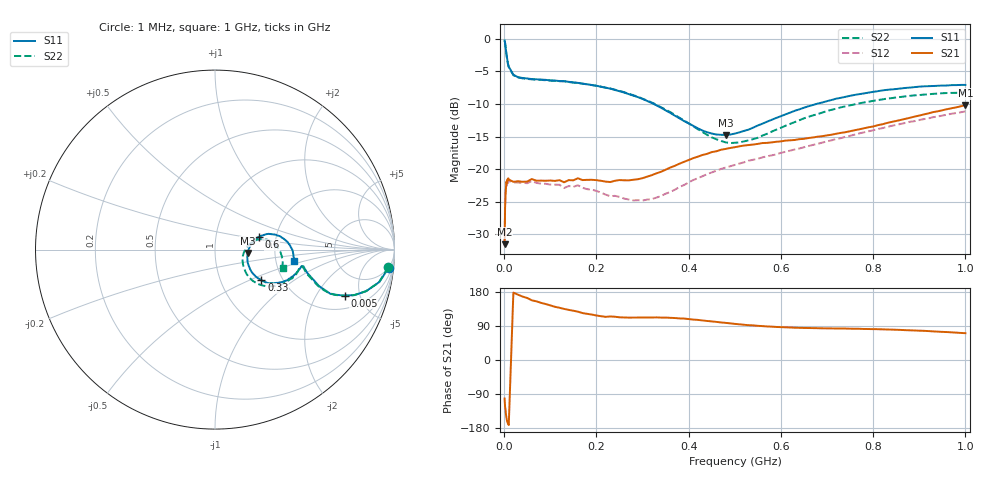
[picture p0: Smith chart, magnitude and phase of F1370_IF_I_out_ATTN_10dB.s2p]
! S-parameters for IF_I+ & IF_I- IDT F1370 DPD Demodulator
! Date Measured:  2015-11-25  RGG
!  Port 1 = Pin 19 = IF_I+
!  Port 2 = Pin 20 = IF_I-
! State: 10 dB attenuation (Gain = Gmax - 10 dB)
! IF Frequency:  1 MHz to 1000 MHz
! RF_INX, RF_INY, IF_Q+, and IF_Q- terminated
! 2300 MHz, 0 dBm signal applied to LO_IN
! Vcc = +5.00 Volts  Icc = approx 275 mA.
! NOTES:  The device was measured on a custom printed circuit evaluation board with individual 50 ohm
!  microstrip lines to the RF and LO pins. The IF outputs are normally connected to balun
!  transformers, which convert the balanced IF output signals to single ended (SE) 50 ohm signals
!  for normal test purposes. For these measurements, to measure the IFI+ and IFI- output SE s-parameters,
!  the chokes associated with the IFI+ and IFI- outputs were removed and a pair of pigtailed
!  50 ohm coaxial lines were soldered to the PCB at these points. 5.00 volt bias was provided
!  to these pins via external bias tees. Data was collected using a calibrated vector
!  network analyzer.  The pigtailed 50 ohm coaxial lines were de-embedded using reference
!  plane extensions. 100 ohm microstrip lines of length 386 mils and 218 mils for the IF_I+ and IF_I-
!  signals, respectively, were de-embedded using Agilent ADS, yielding the reference plane at the IC edge.
!  Only IFI+ and IFI- outputs were measured. IF_Q+ and IF_Q- should be identical.
!  This data is single-ended relative to ports IF_I+ and IF_I- (reference impedance = 50 ohms)
!  Common mode or differential S-parameters may be extracted from this data with a linear simulator.
# mhz S db R 50
! freq  dbS11  angS11  dbS21  angS21  dbS12  angS12  dbS22  angS22
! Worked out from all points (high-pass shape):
!   109 points, 1 MHz to 1 GHz, reference 50 ohm
!   highest |S21| = -10.18 dB at 1 GHz (marker M1); lowest = -31.6 dB at 1 MHz (marker M2)
!   |S21| within 3 dB of the highest: 814.3 MHz to end of sweep
!   lowest |S11| = -14.7 dB at 480 MHz (marker M3), VSWR 1.45, Z = 72.3 - j2.83 ohm
!   |S11| at or under -10 dB: 324.6 MHz to 676.3 MHz (351.8 MHz wide, 70.3 % of centre)
!   |S22| runs from -16.0 to -0.3 dB; largest |S21 - S12| = 0.066
!   S11 on the Smith chart (normalised r, x): 1 MHz: 5, -18; 5 MHz: 2.89, -3.59; 330 MHz: 1.56, -0.59; 600 MHz: 1.63, +0.25; 1 GHz: 2.52, -0.40
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1  -0.24 -5.9  -31.55 -101.9  -31.82 -120.2  -0.27 -5.8
2  -0.60 -11.2  -26.03 -123.1  -25.36 -126.4  -0.61 -11.3
3  -1.17 -15.4  -23.96 -130.1  -23.84 -132.8  -1.18 -15.4
5  -2.31 -19.6  -21.89 -152.1  -22.01 -150.3  -2.37 -19.7
6  -2.80 -20.4  -22.12 -159.3  -22.52 -157.9  -2.91 -20.7
7  -3.23 -21.0  -21.57 -164.2  -21.78 -162.3  -3.35 -20.8
10  -4.27 -19.2  -21.59 -171.5  -21.77 -171.4  -4.32 -19.4
20  -5.50 -14.2  -21.94 177.7  -22.03 178.4  -5.58 -14.5
60  -6.17 -10.8  -21.51 157.5  -21.82 158.6  -6.21 -11.3
130  -6.49 -15.7  -22.02 134.8  -22.89 136.7  -6.50 -16.8
160  -6.75 -18.8  -21.40 127.5  -22.47 129.5  -6.75 -20.4
170  -6.87 -19.6  -21.68 123.9  -22.86 125.6  -6.87 -21.0
280  -8.70 -30.5  -21.63 112.0  -24.80 115.5  -8.64 -33.6
330  -10.19 -33.4  -20.64 112.4  -24.37 122.1  -10.09 -38.2
340  -10.56 -33.5  -20.40 111.9  -24.12 123.5  -10.48 -38.9
430  -14.07 -22.3  -17.82 104.4  -21.08 122.8  -14.30 -32.5
480  -14.73 -5.9  -16.89 98.0  -19.76 118.6  -15.88 -18.2
510  -14.35 3.1  -16.49 94.2  -19.14 115.8  -15.90 -7.7
600  -11.87 16.2  -15.73 86.8  -17.49 109.2  -13.64 11.2
670  -10.13 16.4  -15.13 84.2  -16.27 104.7  -11.73 13.0
840  -7.76 5.2  -12.75 80.2  -13.35 92.6  -9.09 1.2
1000  -7.06 -8.2  -10.18 70.8  -11.12 78.4  -8.19 -15.1
